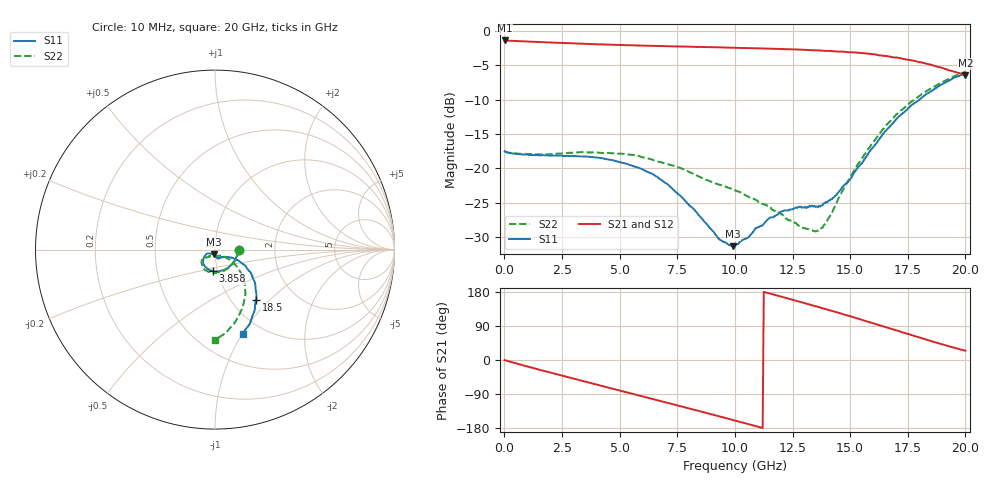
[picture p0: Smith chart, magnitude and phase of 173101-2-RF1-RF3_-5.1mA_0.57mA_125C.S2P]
!  2-Port S-parameters saved by WinCal
! VAR MeasName=S-Parameters (CALIBRATED_DATA) read from VNA (N5242A)
! VAR MeasDate=2017-7-20 10:53:15
! VAR NAME=173101-2-RF1-RF3_-5.1mA_0.57mA_125C
! VAR FILENAME=173101-2-RF1-RF3_-5.1mA_0.57mA_125C.S2P
! VAR DATE=2017-7-20 10:53:15
! VAR PHYS_PORTS=1,2
# Hz S DB R 50
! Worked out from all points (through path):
!   401 points, 10 MHz to 20 GHz, reference 50 ohm
!   highest |S21| = -1.39 dB at 10 MHz (marker M1); lowest = -6.4 dB at 20 GHz (marker M2)
!   group delay of S21, straight-line fit = 46.2 ps
!   lowest |S11| = -31.3 dB at 9.905 GHz (marker M3), VSWR 1.06, Z = 49.2 - j2.56 ohm
!   |S11| at or under -10 dB: start of sweep to 18.01 GHz
!   |S22| runs from -29.2 to -6.0 dB; largest |S21 - S12| = 0.0063
!   S11 on the Smith chart (normalised r, x): 10 MHz: 1.31, -0.01; 3.858 GHz: 0.95, -0.23; 18.5 GHz: 1.29, -0.83; 20 GHz: 0.81, -1.00
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1e7  -17.54 -0.9  -1.39 -0.2  -1.38 -0.2  -17.49 -0.8
1.559225e9  -18.11 -45.0  -1.63 -26.3  -1.63 -26.3  -17.98 -44.2
3.358325e9  -18.28 -87.2  -1.87 -54.8  -1.87 -54.9  -17.65 -84.0
3.858075e9  -18.39 -96.6  -1.93 -62.7  -1.93 -62.7  -17.68 -92.7
5.257375e9  -19.32 -121.9  -2.08 -84.6  -2.09 -84.6  -17.91 -114.8
6.70665e9  -21.47 -139.7  -2.19 -107.3  -2.19 -107.2  -19.06 -130.4
8.4058e9  -26.73 -152.0  -2.32 -134.0  -2.34 -134.0  -21.14 -141.9
9.355325e9  -30.44 -130.2  -2.41 -149.3  -2.40 -149.3  -22.43 -141.7
9.90505e9  -31.35 -105.9  -2.44 -158.1  -2.45 -158.2  -23.08 -140.1
1.0005e10  -31.19 -102.4  -2.46 -159.8  -2.46 -159.8  -23.20 -139.8
1.090455e10  -28.70 -80.7  -2.53 -174.4  -2.54 -174.4  -24.61 -133.0
1.170415e10  -27.02 -75.2  -2.60 172.3  -2.61 172.4  -26.22 -130.5
1.335332e10  -25.45 -63.9  -2.81 144.5  -2.79 144.5  -29.04 -92.0
1.36032e10  -25.69 -57.7  -2.83 140.1  -2.83 140.0  -29.13 -79.1
1.390305e10  -25.08 -52.2  -2.90 135.0  -2.90 135.0  -28.16 -61.0
1.44028e10  -23.92 -40.7  -2.99 126.1  -3.01 126.2  -25.11 -41.7
1.525238e10  -20.25 -26.5  -3.16 110.8  -3.14 110.9  -19.89 -34.4
1.6002e10  -16.89 -25.0  -3.40 96.8  -3.43 96.7  -16.17 -38.1
1.670165e10  -13.97 -29.1  -3.72 83.7  -3.77 83.5  -13.25 -44.4
1.76012e10  -10.99 -38.7  -4.24 67.2  -4.24 67.1  -10.44 -55.6
1.850075e10  -8.81 -51.0  -4.92 50.1  -4.98 50.1  -8.39 -68.5
2e10  -6.16 -71.9  -6.44 24.4  -6.49 24.9  -5.97 -90.0
